DATA_BLOCK DB 103
TITLE =BLOCK DATA FOR SYSTEM BUTTOM TD17
//
AUTHOR : Esposito
FAMILY : TEXER
NAME : SYS_BUTT
VERSION : 0.1


  STRUCT
   COM0 : INT ;
   COM2 : INT ;
   COM4 : INT ;
  END_STRUCT ;
BEGIN
   COM0 := 0;
   COM2 := 0;
   COM4 := 0;
END_DATA_BLOCK

